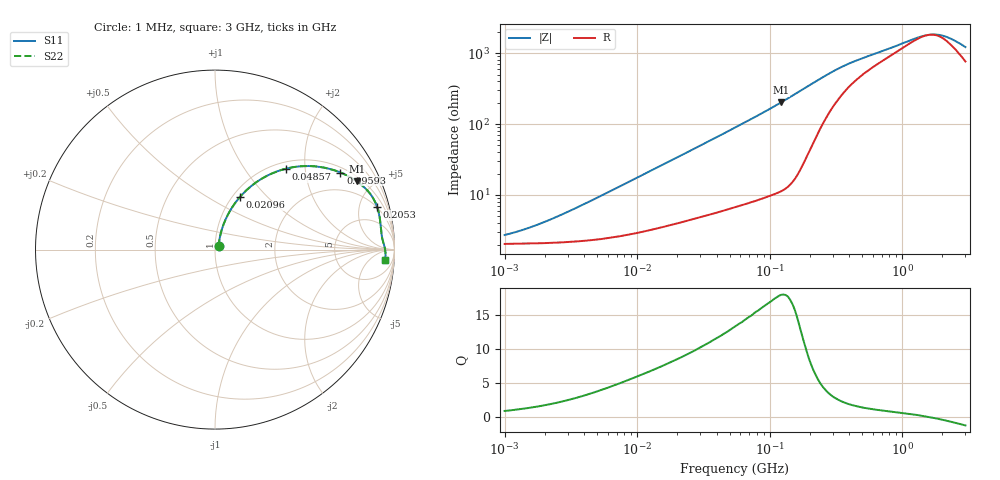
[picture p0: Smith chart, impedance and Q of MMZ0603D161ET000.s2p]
! S-Parameter Data Generated by TDK Corporation
! Copyright(C) 2025 TDK Corporation.
! All Rights Reserved.
! TDK P/N: MMZ0603D161ET000 (Chip Bead)
! Property: |Z|=160ohm at 100MHz
! Size(LxWxT): 0.6x0.3x0.3mm
! Model Type: s2p (Touchstone File Format Version 1.0)
! Frequency: DC=Yes Start=1MHz Stop=3000MHz 202points Log-sweep
! Model Generated on Feb. 6, 2025
! Terms and conditions regarding TDK Simulation Models:
! 1)This simulation model is being provided solely for informational
!  purposes. Please refer to the specifications of the products in
!  terms of detailed characteristics of such products.
! 2)In no event shall TDK Corporation of any of its subsidiaries be
!  liable for any loss or damage arising, directly or indirectly,
!  from any information contained in this simulation model, including,
!  but not limited to loss or damages arising from any inaccuracies,
!  omissions or errors in connection with such information.
! 3)Any and all copyrights on this simulation model are owned by
!  TDK Corporation.  Duplication or redistribution of this simulation
!  model without prior written permission from TDK Corporation
!  is prohibited.
! 4)This simulation model is subject to any modification or change
!  without any prior notice.
! 5)Neither TDK Corporation nor any of its subsidiaries shall make any
!  warranty, express or implied, including but not limited to the
!  correctness, implied warranties of merchantability and fitness for
!  a particular purpose with respect to this simulation models.
! 6)The use of this simulation model shall be deemed to have consented
!  to the terms and conditions hereof.
! Port Assignments:
!  1 ---@@@--- 2
! Applicable Conditions:
!  Temperature = 25 degC
!  DC Bias Current = 0 A
!  Small Signal Operation
# Hz S MA R 50
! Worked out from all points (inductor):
!   201 points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, 1 MHz to 3 GHz, reference 50 ohm
!   read as one part in series: L = 282 nH near 3.9 MHz
!   highest Q = 17.9 at 122 MHz (marker M1), where L = 263 nH
!   self-resonance near 1.593 GHz
!   S11 on the Smith chart (normalised r, x): 1 MHz: 1.04, +0.04; 20.96 MHz: 1.08, +0.70; 48.57 MHz: 1.13, +1.58; 95.93 MHz: 1.19, +3.12; 205.3 MHz: 1.93, +7.22; 3 GHz: 16, -19
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1000000  0.02671 40.5  0.9799 -1.0  0.9799 -1.0  0.02671 40.5
1822989  0.03808 55.8  0.9791 -1.8  0.9791 -1.8  0.03808 55.8
3900413  0.07123 68.2  0.9758 -3.9  0.9758 -3.9  0.07123 68.2
7703107  0.1325 71.4  0.9659 -7.5  0.9659 -7.5  0.1325 71.4
1.461624e7  0.2361 68.6  0.9401 -13.5  0.9401 -13.5  0.2361 68.6
2.095589e7  0.3217 64.8  0.9106 -18.6  0.9106 -18.6  0.3217 64.8
3.254976e7  0.4562 57.6  0.8479 -27.0  0.8479 -27.0  0.4562 57.6
4.857399e7  0.5985 48.8  0.7551 -36.6  0.7551 -36.6  0.5985 48.8
5.477226e7  0.6418 45.9  0.7201 -39.8  0.7201 -39.8  0.6418 45.9
7.248696e7  0.7378 38.7  0.6273 -47.4  0.6273 -47.4  0.7378 38.7
9.593103e7  0.8205 31.6  0.5244 -55.0  0.5244 -55.0  0.8205 31.6
1.219755e8  0.8769 25.7  0.4342 -61.1  0.4342 -61.1  0.8769 25.7
1.614254e8  0.9207 19.4  0.3323 -66.7  0.3323 -66.7  0.9207 19.4
2.052512e8  0.9341 14.8  0.2567 -67.9  0.2567 -67.9  0.9341 14.8
2.136344e8  0.9347 14.1  0.2456 -67.7  0.2456 -67.7  0.9347 14.1
3.741707e8  0.9323 7.1  0.1371 -56.9  0.1371 -56.9  0.9323 7.1
8.005644e8  0.9367 2.9  0.08035 -36.5  0.08035 -36.5  0.9367 2.9
1.347129e9  0.9454 0.7  0.05606 -12.7  0.05606 -12.7  0.9454 0.7
1.712864e9  0.9487 -0.4  0.05166 6.6  0.05166 6.6  0.9487 -0.4
1.931433e9  0.9499 -0.9  0.05263 17.2  0.05263 17.2  0.9499 -0.9
2.177892e9  0.9506 -1.6  0.05627 27.7  0.05627 27.7  0.9506 -1.6
3e9  0.9493 -3.5  0.07786 47.6  0.07786 47.6  0.9493 -3.5
